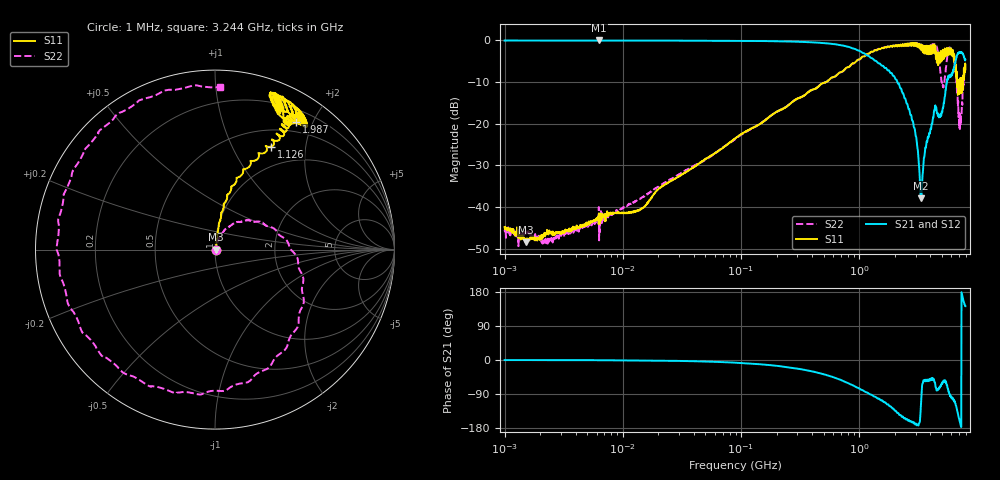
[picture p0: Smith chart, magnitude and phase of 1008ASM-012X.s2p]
!s-Parameter Generated by FASTRON Sdn. Bhd.
!FASTRON P/N : 1008ASM-012X
!Keysight Technologies: E5071C_MY46733604_B.14.02
!Date: Tue Nov 21 11:46:13 2023
!Version  :Rev00  Wed Nov 22 15:30:13 2023
!Data & Calibration Information:
!Freq  S11:SOLT2(ON)  S21:SOLT2(ON)  S12:SOLT2(ON)  S22:SOLT2(ON)
!PortZ  Port1:50+j0  Port2:50+j0
!When reading reference impedance value at option line is always used.
! Remarks : This data is being provided solely for informational purposes.
# Hz S dB R 50
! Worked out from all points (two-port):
!   1599 points, 1 MHz to 7.923 GHz, reference 50 ohm
!   highest |S21| = -0.02 dB at 6.301 MHz (marker M1); lowest = -37.9 dB at 3.345 GHz (marker M2)
!   |S21| within 3 dB of the highest: start of sweep to 1.083 GHz; 7.002 GHz to 7.459 GHz (457.4 MHz wide, 6.33 % of centre)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
!   lowest |S11| = -48.5 dB at 1.505 MHz (marker M3), VSWR 1.01, Z = 50.4 - j0.024 ohm
!   |S11| at or under -10 dB: start of sweep to 522.6 MHz; 6.889 GHz to 6.987 GHz (97.92 MHz wide, 1.41 % of centre); 7.097 GHz to 7.176 GHz (78.67 MHz wide, 1.1 % of centre)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
!   |S22| runs from -49.4 to -0.6 dB; largest |S21 - S12| = 0.013
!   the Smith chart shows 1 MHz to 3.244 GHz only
!   S11 on the Smith chart (normalised r, x): 1 MHz: 1.01, -0.00; 1.126 GHz: 0.71, +1.44; 1.987 GHz: 0.35, +1.77; 3.244 GHz: 0.23, +1.50
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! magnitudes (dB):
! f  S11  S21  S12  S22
! 1 MHz  -44.8  0.0  0.0  -45.5
! 1.505 MHz  -48.5  0.0  0.0  -46.5
! 2.224 MHz  -46.4  0.0  0.0  -47.6
! 4.479 MHz  -44.4  0.0  -0.1  -45.1
! 6.301 MHz  -41.5  0.0  0.0  -48.0
! 13.8 MHz  -40.8  0.0  -0.1  -38.1
! 19.95 MHz  -35.7  -0.1  -0.1  -35.1
! 89.01 MHz  -23.6  -0.1  -0.1  -23.7
! 398.5 MHz  -11.9  -0.5  -0.5  -11.9
! 1.126 GHz  -3.7  -3.3  -3.3  -3.6
! 1.784 GHz  -1.6  -7.2  -7.2  -1.5
! 1.987 GHz  -1.5  -8.7  -8.7  -1.4
! 2.854 GHz  -0.8  -19.5  -19.5  -0.7
! 3.244 GHz  -1.2  -32.0  -32.0  -0.9
! 3.345 GHz  -1.6  -37.9  -37.9  -1.1
! 4.241 GHz  -2.4  -18.6  -18.5  -0.9
! 5.136 GHz  -3.4  -16.2  -16.2  -11.1
! 5.696 GHz  -1.9  -8.9  -8.9  -2.2
! 6.034 GHz  -3.4  -8.3  -8.3  -2.3
! 6.419 GHz  -5.1  -6.0  -6.0  -5.5
! 7.113 GHz  -10.3  -2.9  -2.9  -21.3
! 7.923 GHz  -7.0  -4.6  -4.6  -6.3
